(* Logix 5000 AddOnInstructionDefinition export AMCI_NXFE2_Reset_Errors; software revision 20.03 *)

ADD_ON_INSTRUCTION AMCI_NXFE2_Reset_Errors   (* revision 1.1, vendor AMCI *)
// Revision note:
// Version 1.1 added the slot_axis number and the input parameters can now be tags or discrete values.
VAR_INPUT
   slot_number : INT; {required}
END_VAR
VAR_IN_OUT
   NXFE2_output_data : _000A:NXFE2_0986AEB4:O:0; {required}
END_VAR
VAR
   command_data_block : INT[10];
        [0]   // Command Bits MSW
        [1]   // Command Bits LSW
        [2]   // Upper Target Position
        [3]   // Lower Target Position
        [4]   // Upper Programmed Speed
        [5]   // Lower Programmed Speed
END_VAR

ROUTINE Logic   (* ladder *)
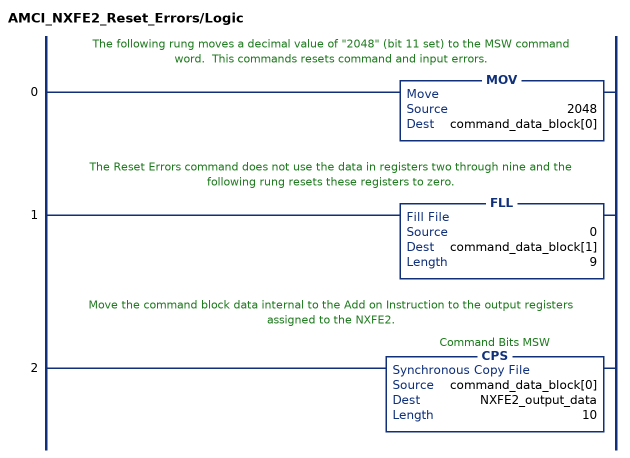
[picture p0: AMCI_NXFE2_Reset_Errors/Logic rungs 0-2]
   // The following rung moves a decimal value of "2048" (bit 11 set) to the MSW command word.  This commands resets command and input errors.
   0: MOV(2048,command_data_block[0]);
   // The Reset Errors command does not use the data in registers two through nine and the following rung resets these registers to zero.
   1: FLL(0,command_data_block[1],9);
   // Move the command block data internal to the Add on Instruction to the output registers assigned to the NXFE2.
   2: CPS(command_data_block[0],NXFE2_output_data,10);
END_ROUTINE
END_ADD_ON_INSTRUCTION
